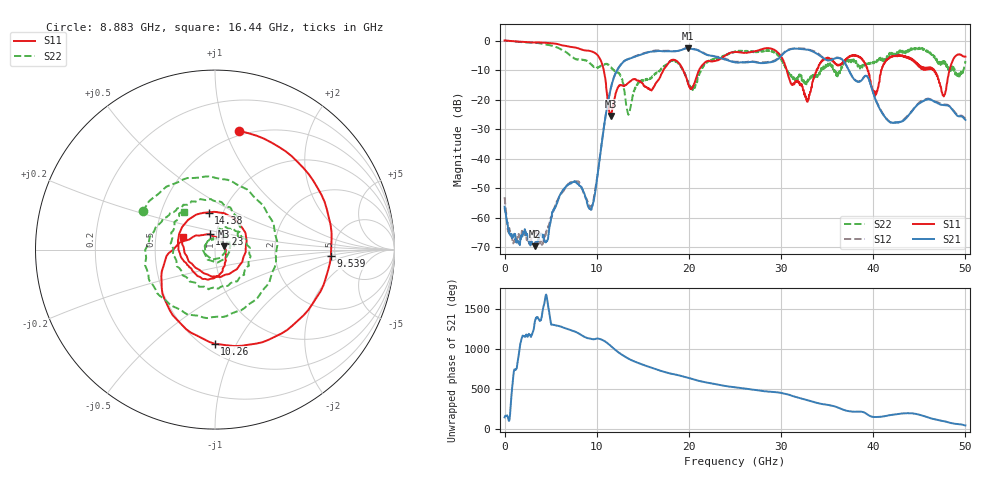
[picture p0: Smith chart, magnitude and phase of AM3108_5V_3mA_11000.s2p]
# Hz S DB R 50.0
!freq dBS11 angS11 dBS21 angS21 dBS12 angS12 dBS22 angS22
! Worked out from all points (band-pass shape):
!   1601 points, 10 MHz to 50 GHz, reference 50 ohm
!   highest |S21| = -2.62 dB at 19.91 GHz (marker M1); lowest = -69.6 dB at 3.259 GHz (marker M2)
!   |S21| within 3 dB of the highest: 14 GHz to 23.05 GHz (9.048 GHz wide, 48.8 % of centre); 29.89 GHz to 34.42 GHz (4.525 GHz wide, 14.1 % of centre)
!   lowest |S11| = -25.5 dB at 11.51 GHz (marker M3), VSWR 1.11, Z = 55.2 + j2.03 ohm
!   |S11| at or under -10 dB: 10.76 GHz to 17.25 GHz (6.485 GHz wide, 46.3 % of centre); 19.38 GHz to 21.11 GHz (1.723 GHz wide, 8.51 % of centre); 30.62 GHz to 33.85 GHz (3.23 GHz wide, 10 % of centre)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
!   |S22| runs from -25.1 to 0.0 dB; largest |S21 - S12| = 0.027
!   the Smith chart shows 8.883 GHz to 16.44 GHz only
!   S11 on the Smith chart (normalised r, x): 8.883 GHz: 0.46, +1.11; 9.539 GHz: 4.59, -0.56; 10.26 GHz: 0.57, -0.82; 11.23 GHz: 0.93, +0.16; 14.38 GHz: 0.86, +0.37; 16.44 GHz: 0.69, +0.10
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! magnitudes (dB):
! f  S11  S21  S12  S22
! 10 MHz  0.0  -56.3  -53.1  0.0
! 978.6 MHz  -0.2  -66.1  -68.3  -0.3
! 3.259 GHz  -0.7  -69.6  -63.8  -0.8
! 8.352 GHz  -3.0  -49.8  -49.8  -6.4
! 8.883 GHz  -3.4  -53.8  -53.5  -6.8
! 9.539 GHz  -3.8  -56.0  -55.5  -8.4
! 10.26 GHz  -5.6  -41.6  -41.5  -8.9
! 11.23 GHz  -20.9  -20.9  -20.7  -8.1
! 11.51 GHz  -25.5  -16.5  -16.4  -9.0
! 13.44 GHz  -14.3  -6.3  -6.2  -25.1
! 14.38 GHz  -13.6  -5.2  -5.0  -14.8
! 16.44 GHz  -14.4  -3.6  -3.3  -11.2
! 16.69 GHz  -13.3  -3.5  -3.3  -10.8
! 18.38 GHz  -6.5  -3.6  -3.6  -7.0
! 19.91 GHz  -14.8  -2.6  -2.6  -13.9
! 25 GHz  -3.9  -7.4  -7.2  -3.9
! 33.35 GHz  -15.6  -3.5  -3.4  -12.7
! 38 GHz  -4.9  -13.4  -13.3  -6.6
! 40.22 GHz  -18.7  -19.8  -19.6  -7.6
! 41.69 GHz  -6.0  -27.3  -27.2  -5.2
! 47.66 GHz  -18.9  -21.9  -21.6  -7.7
! 50 GHz  -5.5  -26.9  -26.4  -6.9
